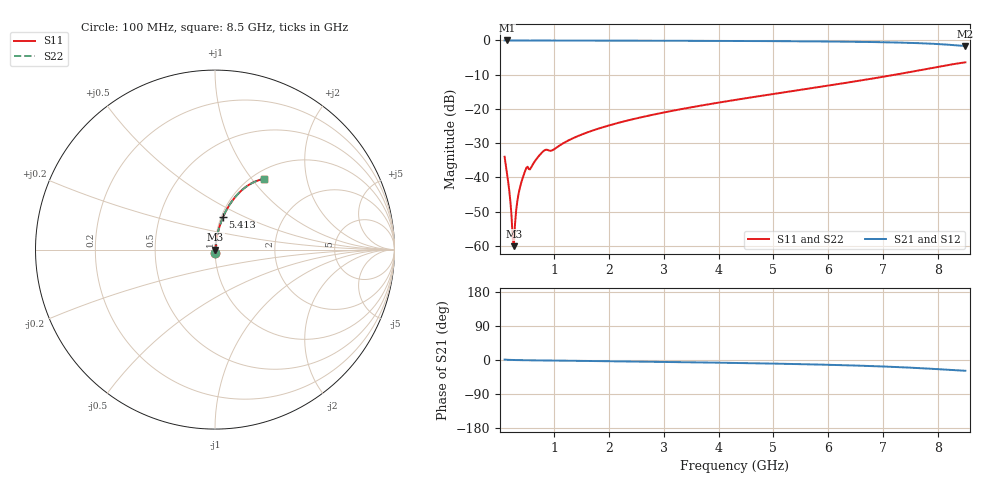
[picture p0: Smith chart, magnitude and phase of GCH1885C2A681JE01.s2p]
!Murata Part Number: GCH1885C2A681JE01
!These Parameters are Measured in Series Mode Connection
!Data Generated on Jun 19, 2026
!  o--ll--o
!Port1  Port2
!  o------o
!Operation Temp=25[degC], DC Bias Voltage=0[V]
!Freq. Start=100[MHz] Stop=9[GHz] 401[Steps]
# Hz S RI R 50
!Freq.(Hz) S11(Real) S11(Imag) S21(Real) S21(Imag) S12(Real) S12(Imag) S22(Real) S22(Imag)
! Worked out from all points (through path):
!   401 points, 100 MHz to 8.5 GHz, reference 50 ohm
!   highest |S21| = -0.01 dB at 142 MHz (marker M1); lowest = -1.6 dB at 8.5 GHz (marker M2)
!   group delay of S21, straight-line fit = 8.19 ps
!   lowest |S11| = -60.1 dB at 268 MHz (marker M3), VSWR 1.00, Z = 50.1 + j0.0439 ohm
!   |S11| at or under -10 dB: start of sweep to 7.223 GHz
!   |S22| runs from -60.1 to -6.4 dB; largest |S21 - S12| = 0
!   S11 on the Smith chart (normalised r, x): 100 MHz: 1.00, -0.04; 5.413 GHz: 1.02, +0.38; 8.5 GHz: 1.12, +1.15
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1e8  0.000992 -0.02  0.999 0.02  0.999 0.02  0.000992 -0.02
1.42e8  0.000776 -0.0116  0.9992 0.0116  0.9992 0.0116  0.000776 -0.0116
1.84e8  0.000747 -0.00643  0.9993 0.00643  0.9993 0.00643  0.000747 -0.00643
2.26e8  0.000794 -0.00263  0.9992 0.00263  0.9992 0.00263  0.000794 -0.00263
2.47e8  0.000835 -0.00103  0.9992 0.00103  0.9992 0.00103  0.000835 -0.00103
2.68e8  0.000885 0.000438  0.9991 -0.000438  0.9991 -0.000438  0.000885 0.000438
2.89e8  0.000945 0.0018  0.9991 -0.0018  0.9991 -0.0018  0.000945 0.0018
3.31e8  0.00109 0.0043  0.9989 -0.0043  0.9989 -0.0043  0.00109 0.0043
3.73e8  0.00128 0.00662  0.9987 -0.00662  0.9987 -0.00662  0.00128 0.00662
4.36e8  0.00175 0.00999  0.9982 -0.00999  0.9982 -0.00999  0.00175 0.00999
4.99e8  0.0036 0.0134  0.9964 -0.0134  0.9964 -0.0134  0.0036 0.0134
5.83e8  0.0031 0.0136  0.9969 -0.0136  0.9969 -0.0136  0.0031 0.0136
8.14e8  0.00562 0.0237  0.9944 -0.0237  0.9944 -0.0237  0.00562 0.0237
9.82e8  0.00582 0.0245  0.9942 -0.0245  0.9942 -0.0245  0.00582 0.0245
1.507e9  0.00591 0.0419  0.9941 -0.0419  0.9941 -0.0419  0.00591 0.0419
2.116e9  0.00877 0.0601  0.9912 -0.0601  0.9912 -0.0601  0.00877 0.0601
2.914e9  0.0136 0.0847  0.9864 -0.0847  0.9864 -0.0847  0.0136 0.0847
4.3e9  0.0265 0.1325  0.9735 -0.1325  0.9735 -0.1325  0.0265 0.1325
5.413e9  0.0443 0.1802  0.9557 -0.1802  0.9557 -0.1802  0.0443 0.1802
5.707e9  0.0509 0.195  0.9491 -0.195  0.9491 -0.195  0.0509 0.195
7.114e9  0.107 0.286  0.893 -0.286  0.893 -0.286  0.107 0.286
8.5e9  0.2716 0.3943  0.7284 -0.3943  0.7284 -0.3943  0.2716 0.3943
